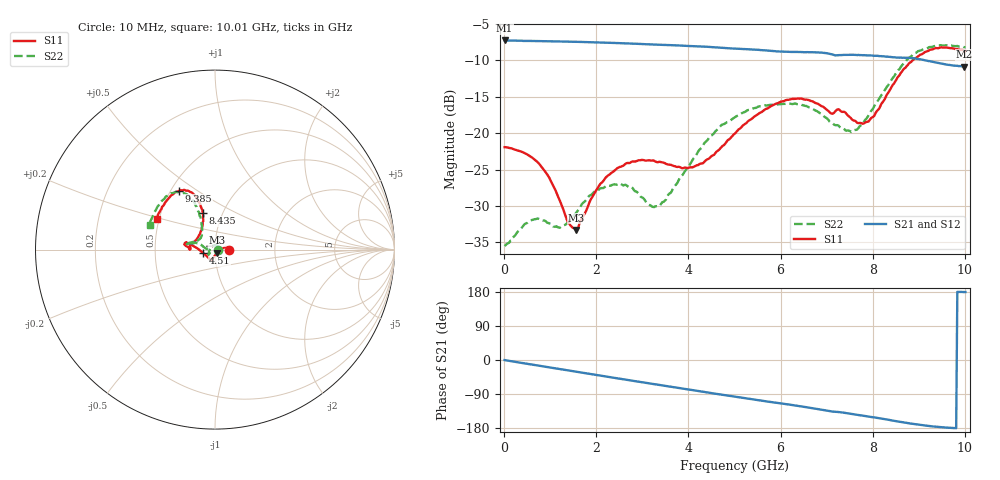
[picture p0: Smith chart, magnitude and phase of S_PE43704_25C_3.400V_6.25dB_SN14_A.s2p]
! Device ID: PE43704
! Dir: z:\PE43704\PE43704_Char_1_20130516\PE43704\AMB\3p400V\6p25dB
! Serial: 14
! Insertion: A
! Impedance: 50 ohm
! Temp: Amb
! VDD: 3.400V
! Attenuation Step: 6.25dB
! IDD: 1.140292e-01mA
#  Hz  S  RI  R  50
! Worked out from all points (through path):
!   401 points, 10 MHz to 10.01 GHz, reference 50 ohm
!   highest |S21| = -7.26 dB at 10 MHz (marker M1); lowest = -10.8 dB at 9.985 GHz (marker M2)
!   group delay of S21, straight-line fit = 51.6 ps
!   lowest |S11| = -33.3 dB at 1.56 GHz (marker M3), VSWR 1.04, Z = 51.3 - j1.75 ohm
!   |S11| at or under -10 dB: start of sweep to 8.861 GHz
!   |S22| runs from -35.5 to -7.9 dB; largest |S21 - S12| = 0.0031
!   S11 on the Smith chart (normalised r, x): 10 MHz: 1.17, +0.00; 4.51 GHz: 0.87, -0.03; 8.435 GHz: 0.81, +0.34; 9.385 GHz: 0.55, +0.42; 10.01 GHz: 0.48, +0.19
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1e7  0.0802 1.28e-05  0.4336 -0.00161  0.4339 -0.0016  0.0167 0.000514
7.6e8  0.0599 0.0146  0.4142 -0.1124  0.4142 -0.1123  0.0035 0.0255
1.21e9  0.0343 0.000905  0.3898 -0.1739  0.3899 -0.1738  -0.0153 0.0164
1.41e9  0.0219 -0.0098  0.3758 -0.1995  0.3758 -0.1994  -0.0237 0.00781
1.56e9  0.0133 -0.017  0.3643 -0.218  0.3643 -0.2178  -0.0284 0.000412
1.685e9  0.0069 -0.025  0.3537 -0.2331  0.3537 -0.2328  -0.032 -0.0059
2.06e9  -0.00779 -0.043  0.3185 -0.2737  0.3185 -0.2736  -0.0359 -0.02
2.435e9  -0.0161 -0.0545  0.2788 -0.3089  0.2789 -0.309  -0.0359 -0.0259
3.36e9  -0.0259 -0.058  0.1673 -0.3694  0.1678 -0.3691  -0.03 -0.00967
4.035e9  -0.0447 -0.0374  0.0792 -0.3889  0.0797 -0.3889  -0.0599 0.0128
4.51e9  -0.0675 -0.018  0.0166 -0.39  0.0167 -0.3902  -0.0911 0.0332
5.01e9  -0.0993 0.00703  -0.0448 -0.3784  -0.0445 -0.3786  -0.1241 0.0344
5.96e9  -0.1573 0.0394  -0.1465 -0.3339  -0.1454 -0.3341  -0.1541 0.0347
6.685e9  -0.1646 0.022  -0.2172 -0.2868  -0.2172 -0.2868  -0.1427 0.0369
7.585e9  -0.1132 0.0462  -0.2766 -0.2072  -0.2761 -0.2071  -0.0778 0.0702
7.935e9  -0.0823 0.0921  -0.2956 -0.1726  -0.2958 -0.173  -0.0724 0.1172
8.36e9  -0.0663 0.1837  -0.3104 -0.1243  -0.3099 -0.1258  -0.0881 0.2019
8.435e9  -0.0684 0.2037  -0.3122 -0.1154  -0.3116 -0.1157  -0.0968 0.2194
8.86e9  -0.1081 0.2969  -0.3209 -0.0667  -0.3187 -0.0676  -0.1559 0.3073
9.385e9  -0.2022 0.3268  -0.3046 -0.0204  -0.3053 -0.0191  -0.255 0.3053
9.985e9  -0.3204 0.1824  -0.287 0.00326  -0.2882 0.00422  -0.3608 0.1463
1.001e10  -0.3255 0.1718  -0.288 0.00328  -0.2894 0.00411  -0.3644 0.1377
